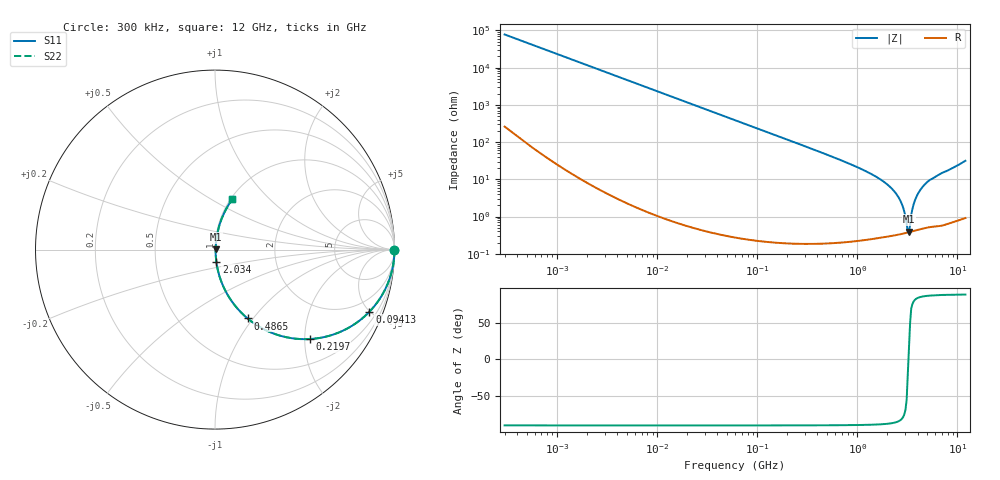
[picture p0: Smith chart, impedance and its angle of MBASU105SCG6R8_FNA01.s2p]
! MBASU105SCG6R8_FNA01  S-PARAMETER MODEL  ( Standard Model )
! Model Generated by TAIYO YUDEN Corporation (http://www.ty-top.com)
! Version 1.0
! TAIYO YUDEN Control No. 230609
! Copyright(c) 2023 TAIYO YUDEN CO.,LTD. All Rights Reserved.
! Product Description (link to TY-COMPAS)
! https://ds.yuden.co.jp/TYCOMPAS/or/detail?pn=MBASU105SCG6R8DFNA01&u=M
! Products Name : Multilayer Ceramic Capacitors
! Characteristics :
!  Capacitance : 6.8 [pF] , Rated Voltage : 50 [V] , TCC : CG / C0G
!  Case Size : 1.0 x 0.5 / 0.039 x 0.02 [mm/inch] , Thickness : 0.5 / 0.02 [mm/inch]
!  (Conditions: Temperature = 25 [degC] , DC Bias Voltage = 0 [V])
! External Node Assignments :
!  1  o---| |---o  2
! GND o---------o GND
! Frequency Range : 0.3MHz  -  12000MHz  [ 401 STEP ]
# MHZ S RI R 50
! Freq[MHz].  S11 Real  S11 Imag  S21 Real  S21 Imag  S12 Real  S12 Imag  S22 Real  S22 Imag
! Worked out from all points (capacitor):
!   401 points, 300 kHz to 12 GHz, reference 50 ohm
!   read as one part in series: C = 6.8 pF near 316.3 kHz
!   lowest |Z| = 394 mohm at 3.277 GHz (marker M1)
!   series resonance near 3.238 GHz, so ESL is about 360 pH
!   S11 on the Smith chart (normalised r, x): 300 kHz: open; 94.13 MHz: 1.00, -4.97; 219.7 MHz: 1.00, -2.12; 486.5 MHz: 1.00, -0.94; 2.034 GHz: 1.01, -0.14; 12 GHz: 1.02, +0.63
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0.3  1 -0.00128  5.93e-06 0.00128  5.93e-06 0.00128  1 -0.00128
1.769972  0.9999 -0.00756  6.27e-05 0.00756  6.27e-05 0.00756  0.9999 -0.00756
10.44266  0.998 -0.0445  0.00201 0.0445  0.00201 0.0445  0.998 -0.0445
60  0.9381 -0.2405  0.0619 0.2405  0.0619 0.2405  0.9381 -0.2405
94.13233  0.8603 -0.3462  0.1397 0.3462  0.1397 0.3462  0.8603 -0.3462
219.7372  0.5291 -0.4983  0.4709 0.4983  0.4709 0.4983  0.5291 -0.4983
353.9943  0.2996 -0.4567  0.7004 0.4567  0.7004 0.4567  0.2996 -0.4567
486.4723  0.182 -0.3839  0.818 0.3839  0.818 0.3839  0.182 -0.3839
1166.079  0.0316 -0.1685  0.9684 0.1685  0.9684 0.1685  0.0316 -0.1685
2033.931  0.00762 -0.0685  0.9924 0.0685  0.9924 0.0685  0.00762 -0.0685
2088.533  0.0071 -0.0643  0.9929 0.0643  0.9929 0.0643  0.0071 -0.0643
2650.866  0.00411 -0.0283  0.9959 0.0283  0.9959 0.0283  0.00411 -0.0283
2870.14  0.00374 -0.0167  0.9963 0.0167  0.9963 0.0167  0.00374 -0.0167
3107.553  0.00366 -0.00521  0.9963 0.00521  0.9963 0.00521  0.00366 -0.00521
3190.978  0.0037 -0.00134  0.9963 0.00134  0.9963 0.00134  0.0037 -0.00134
3276.641  0.00377 0.00111  0.9962 -0.00111  0.9962 -0.00111  0.00377 0.00111
3364.605  0.00386 0.00452  0.9961 -0.00452  0.9961 -0.00452  0.00386 0.00452
3642.919  0.00448 0.0204  0.9955 -0.0204  0.9955 -0.0204  0.00448 0.0204
3841.137  0.00517 0.0308  0.9948 -0.0308  0.9948 -0.0308  0.00517 0.0308
4623.766  0.00941 0.0677  0.9906 -0.0677  0.9906 -0.0677  0.00941 0.0677
6524.734  0.0226 0.1295  0.9774 -0.1295  0.9774 -0.1295  0.0226 0.1295
12000  0.0969 0.2818  0.9031 -0.2818  0.9031 -0.2818  0.0969 0.2818
